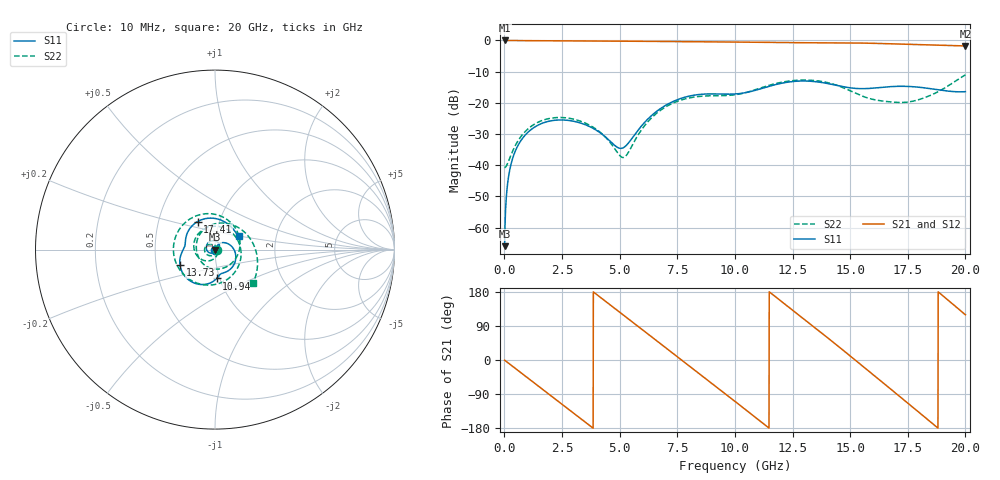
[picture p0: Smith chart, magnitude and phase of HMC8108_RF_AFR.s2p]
! Analog Devices, Inc.
! 1 Analog Way
! Wilmington, MA 01887
! http://www.analog.com
! Date:  2021-09-07 NN
! Board Name:  EV1HMC8108LC5 Revision A with HMC8108LC5 installed
! File Description:  Automatic Fixture Removal S-Parameters for RF Port connector and board loss de-embedding
! File Generation:  Calibrated Network Analyzer
! Chip Part Number:  HMC8108
! Chip Description:  X-Band, GaAs, MMIC, Low Noise Converter
! Chip Frequency:  9 to 10 GHz
! Chip Package:  LCC, 5 x 5 x 1.12 mm
! RF Port:  HMC8108LC5 removed and end of trace left open
! Note:
!  Analog Devices supplies this data as a sample of measured data at the evaluation board
!  ports for this product.  Your particular data for this product may vary.
!  Analog Devices reserves the right to change this data at anytime.
!  All lines below in this file are as is from the Network Analyzer.
!Agilent Technologies,N5245A,MY52451809,A.10.47.06
!Automatic Fixture Removal (AFR)
!Date: Friday, August 27, 2021 5:23:10 AM
!S2P File: Measurements: S11,S21,S12,S22:
# MHz S  RI  R 50
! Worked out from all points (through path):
!   2000 points, 10 MHz to 20 GHz, reference 50 ohm
!   highest |S21| = 0.00 dB at 10 MHz (marker M1); lowest = -1.8 dB at 20 GHz (marker M2)
!   group delay of S21, straight-line fit = 133 ps
!   lowest |S11| = -66.0 dB at 10 MHz (marker M3), VSWR 1.00, Z = 50 - j0.0367 ohm
!   |S11| at or under -10 dB: start of sweep to end of sweep
!   |S22| runs from -40.8 to -11.0 dB; largest |S21 - S12| = 1.4e-15
!   S11 on the Smith chart (normalised r, x): 10 MHz: 1.00, -0.00; 10.94 GHz: 0.97, -0.32; 13.73 GHz: 0.66, -0.12; 17.41 GHz: 0.79, +0.26; 20 GHz: 1.29, +0.19
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10  0.000344 -0.000367  1 -0.00817  1 -0.00817  0.00913 -0.000466
250  -0.00189 -0.00882  0.9778 -0.2025  0.9778 -0.2025  0.00718 -0.0114
780  -0.0181 -0.0197  0.7997 -0.5918  0.7997 -0.5918  -0.0081 -0.0297
2040  -0.0475 0.0203  -0.0923 -0.9828  -0.0923 -0.9828  -0.0545 -0.0163
3350  0.00678 0.0464  -0.9006 -0.3912  -0.9006 -0.3912  -0.0423 0.0267
4220  0.0248 0.0198  -0.9352 0.2894  -0.9352 0.2894  -0.0127 0.0296
5160  0.013 0.0139  -0.4692 0.8546  -0.4692 0.8546  0.0126 0.00417
5910  0.024 0.0332  0.109 0.964  0.109 0.964  0.00929 -0.034
6680  0.0682 0.0346  0.6528 0.7089  0.6528 0.7089  -0.0344 -0.0627
7420  0.1088 -0.00646  0.9336 0.2086  0.9336 0.2086  -0.0948 -0.0399
8140  0.1122 -0.0673  0.8861 -0.3437  0.8861 -0.3437  -0.1175 0.0338
9130  0.0674 -0.1216  0.3577 -0.8747  0.3577 -0.8747  -0.0278 0.127
10010  0.0335 -0.1346  -0.3136 -0.8885  -0.3136 -0.8885  0.112 0.0748
10940  0.00973 -0.1604  -0.8408 -0.4134  -0.8408 -0.4134  0.1182 -0.1149
12020  -0.0672 -0.1947  -0.8371 0.397  -0.8371 0.397  -0.1112 -0.1822
13340  -0.1837 -0.1232  -0.0259 0.9183  -0.0259 0.9183  -0.2109 0.0911
13730  -0.1954 -0.0845  0.2708 0.8774  0.2708 0.8774  -0.1468 0.1657
15200  -0.1702 0.0131  0.913 0.0133  0.913 0.0133  0.1392 0.0385
16670  -0.1506 0.1002  0.2703 -0.8442  0.2703 -0.8442  -0.0567 -0.0873
17410  -0.0965 0.1565  -0.2864 -0.822  -0.2864 -0.822  -0.1011 -0.0139
18710  0.0514 0.1557  -0.8387 -0.0791  -0.8387 -0.0791  0.000497 0.1439
20000  0.1321 0.0733  -0.4 0.7123  -0.4 0.7123  0.2127 -0.1848
